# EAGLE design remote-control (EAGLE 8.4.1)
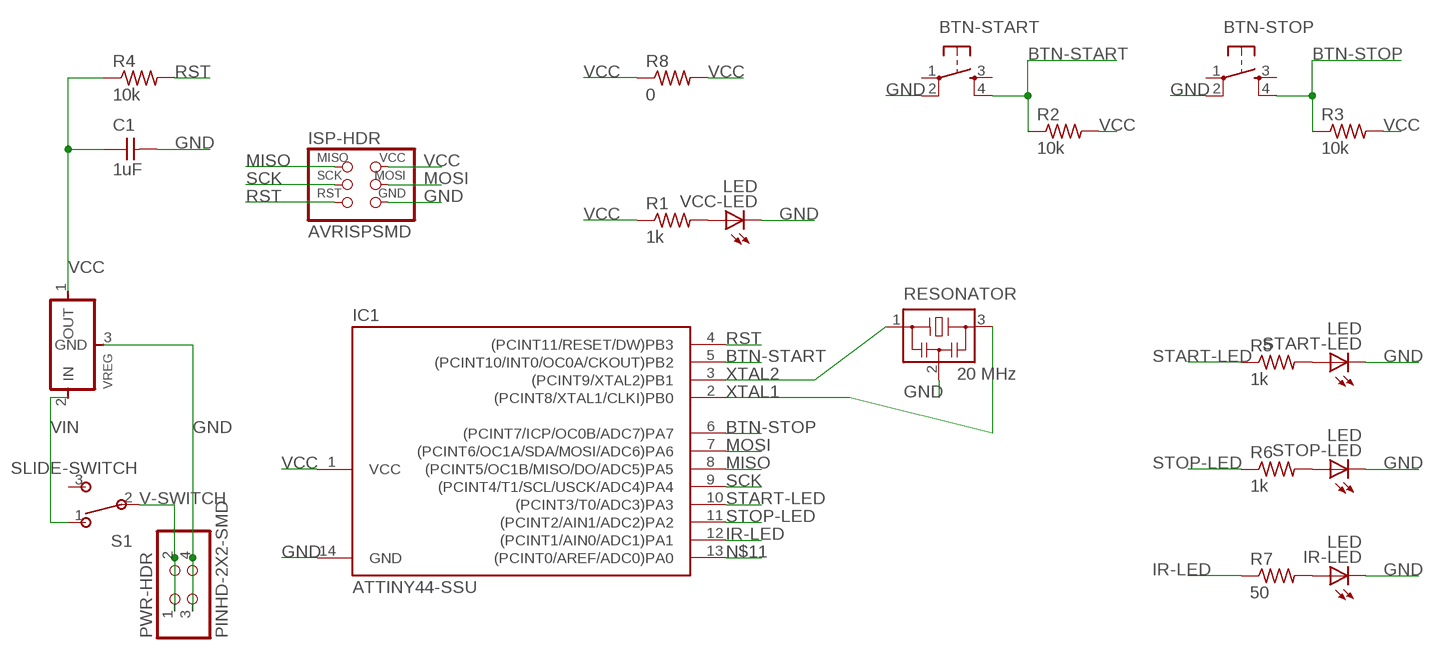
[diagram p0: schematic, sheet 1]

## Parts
BTN-START  6MM_SWITCH6MM_SWITCH  [6MM_SWITCH]
BTN-STOP  6MM_SWITCH6MM_SWITCH  [6MM_SWITCH]
C1  1uF  CAP-UNPOLARIZEDFAB  [C1206FAB]
IC1  ATTINY44-SSU  [SOIC14]
IR-LED  LED  [LED1206]
ISP-HDR  AVRISPSMD  [2X03SMD]
PWR-HDR  PINHD-2X2-SMD  [2X02SMD]
R1  1k  RES-US1206FAB  [R1206FAB]
R2  10k  RES-US1206FAB  [R1206FAB]
R3  10k  RES-US1206FAB  [R1206FAB]
R4  10k  RES-US1206FAB  [R1206FAB]
R5  1k  RES-US1206FAB  [R1206FAB]
R6  1k  RES-US1206FAB  [R1206FAB]
R7  50  RES-US1206FAB  [R1206FAB]
R8  0  RES-US1206FAB  [R1206FAB]
RESONATOR  20 MHz  RESONATOR  [EFOBM]
S1  SLIDE-SWITCH  [AYZ0102AGRLC]
START-LED  LED  [LED1206]
STOP-LED  LED  [LED1206]
VCC-LED  LED  [LED1206]
VREG  REGULATORSOT23  [SOT23]

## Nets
BTN-START: BTN-START.4(S1) IC1.5((PCINT10/INT0/OC0A/CKOUT)PB2) R2.1
BTN-STOP: BTN-STOP.4(S1) IC1.6((PCINT7/ICP/OC0B/ADC7)PA7) R3.1
GND: BTN-START.2(P1) BTN-STOP.2(P1) C1.2 IC1.14(GND) IR-LED.2(C) ISP-HDR.6(GND) PWR-HDR.3 PWR-HDR.4 RESONATOR.2 START-LED.2(C) STOP-LED.2(C) VCC-LED.2(C) VREG.3(GND)
IR-LED: IC1.12((PCINT1/AIN0/ADC1)PA1) R7.1
MISO: IC1.8((PCINT5/OC1B/MISO/DO/ADC5)PA5) ISP-HDR.1(MISO)
MOSI: IC1.7((PCINT6/OC1A/SDA/MOSI/ADC6)PA6) ISP-HDR.4(MOSI)
N$2: R5.2 START-LED.1(A)
N$3: R6.2 STOP-LED.1(A)
N$4: IR-LED.1(A) R7.2
N$9: R1.2 VCC-LED.1(A)
N$11: IC1.13((PCINT0/AREF/ADC0)PA0)
RST: IC1.4((PCINT11/RESET/DW)PB3) ISP-HDR.5(RST) R4.2
SCK: IC1.9((PCINT4/T1/SCL/USCK/ADC4)PA4) ISP-HDR.3(SCK)
START-LED: IC1.10((PCINT3/T0/ADC3)PA3) R5.1
STOP-LED: IC1.11((PCINT2/AIN1/ADC2)PA2) R6.1
V-SWITCH: PWR-HDR.1 PWR-HDR.2 S1.2
VCC: C1.1 IC1.1(VCC) ISP-HDR.2(VCC) R1.1 R2.2 R3.2 R4.1 R8.1 R8.2 VREG.1(OUT)
VIN: S1.1 VREG.2(IN)
XTAL1: IC1.2((PCINT8/XTAL1/CLKI)PB0) RESONATOR.3
XTAL2: IC1.3((PCINT9/XTAL2)PB1) RESONATOR.1
Unconnected: BTN-START.1(P) BTN-START.3(S) BTN-STOP.1(P) BTN-STOP.3(S) S1.3

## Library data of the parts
BTN-START BTN-STOP = fab:6MM_SWITCH: OMRON SWITCH
C1 = fab:CAP-UNPOLARIZED
IC1 = fab:ATTINY44
IR-LED START-LED STOP-LED VCC-LED = fab:LED: LED
ISP-HDR = fab:AVRISP
PWR-HDR = fab:PINHD-2X2-SMD
R1-R8 = fab:RES-US: Resistor (US Symbol)
RESONATOR = fab:RESONATOR
S1 = fab:SLIDE-SWITCH: SMD slide-switch AYZ0102AGRLC as found in the fablab inventory. Includes the mounting holes. Made by Zaerc.
VREG = fab:REGULATOR

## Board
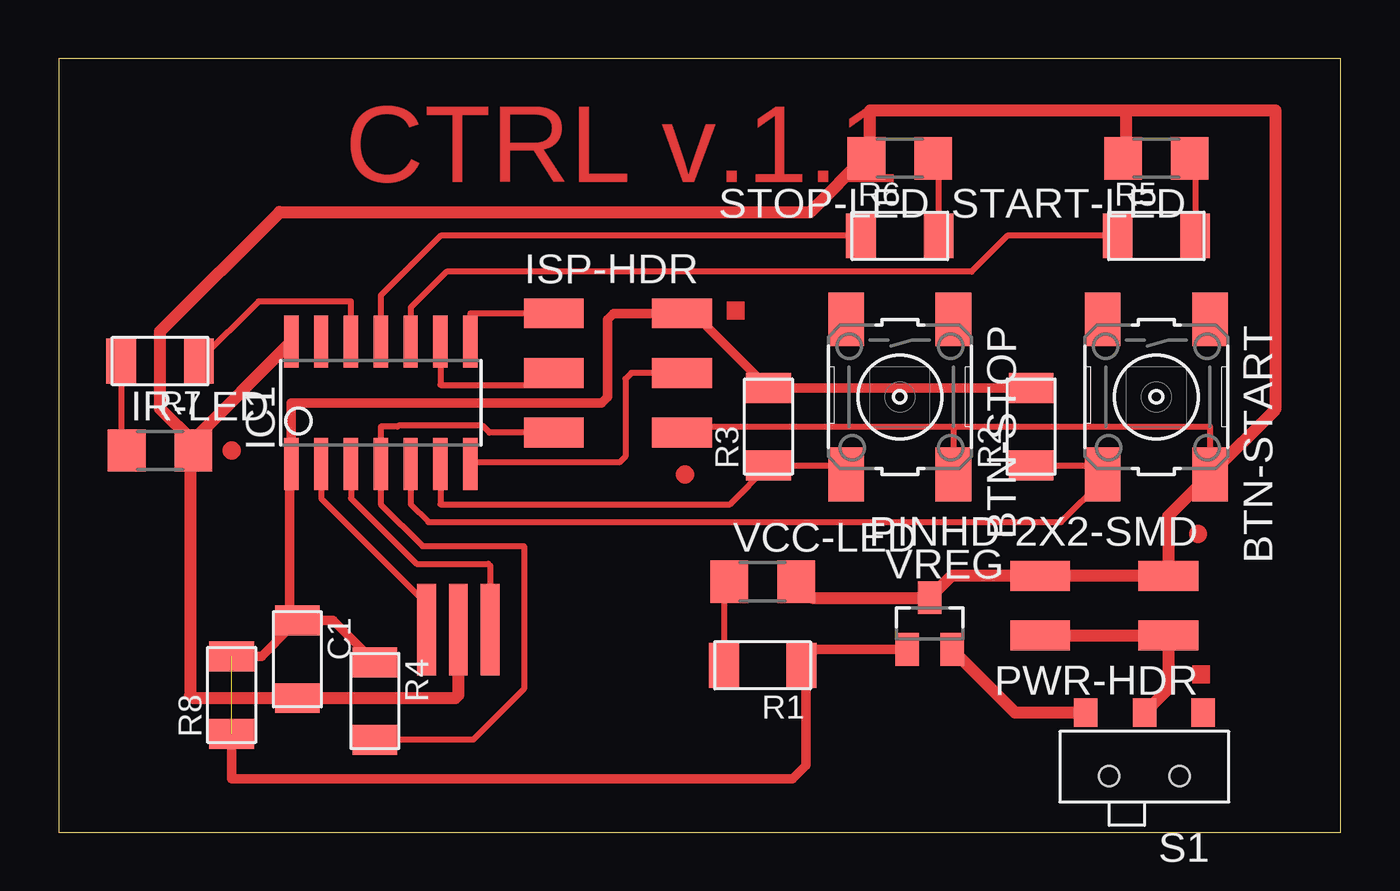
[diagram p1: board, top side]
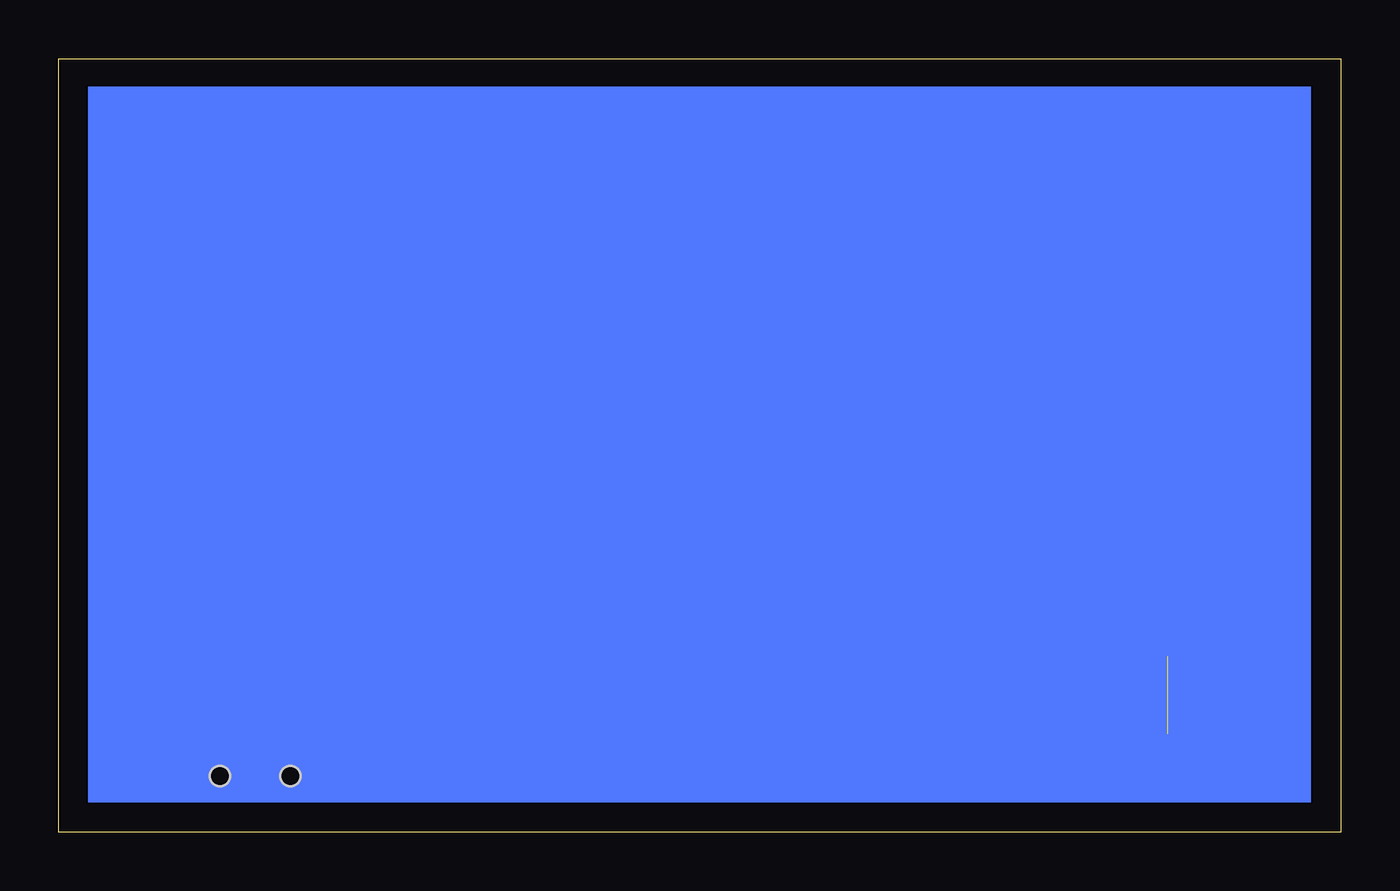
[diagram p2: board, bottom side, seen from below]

Size 54.59 x 32.94 mm. Coordinates in mm from the lower left corner, seen from the top.
Outline: 0,0 54.59,0 54.59,32.94 0,32.94 0,0
Copper layers (1*16): Top 0.035mm / dielectric 1.5mm / Bottom 0.035mm
Design rules "default *": minimum track width 0.000253125mm, minimum drill 0.35mm, track to track 15.625mil, track to pad 15.625mil, pad to pad 15.625mil, via to via 15.625mil, smd to smd 6mil, copper to edge 15.625mil, drill to drill 15.625mil, minimum pad ring 10mil, minimum via ring 8mil, stop-mask expansion 4mil, vias tented up to drill 0mil, thermal gap 10mil

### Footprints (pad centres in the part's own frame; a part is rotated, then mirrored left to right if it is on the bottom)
6MM_SWITCH = smd 2.286 x 1.524: 1 -3.302,2.286; 2 3.302,2.286; 3 -3.302,-2.286; 4 3.302,-2.286
C1206FAB = smd 1.27 x 1.905: 1 -1.651,0; 2 1.651,0
SOIC14 = smd 0.61 x 2.21: 1 -3.81,-2.603; 2 -2.54,-2.603; 3 -1.27,-2.603; 4 0,-2.603; 5 1.27,-2.603; 6 2.54,-2.603; 7 3.81,-2.603; 8 3.81,2.603; 9 2.54,2.603; 10 1.27,2.603; 11 0,2.603; 12 -1.27,2.603; 13 -2.54,2.603; 14 -3.81,2.603
LED1206 = smd 1.6 x 1.803: 1 -1.422,0; 2 1.422,0
2X03SMD = smd 2.54 x 1.27: 1 -2.54,2.54; 2 2.92,2.54; 3 -2.54,0; 4 2.92,0; 5 -2.54,-2.54; 6 2.92,-2.54
2X02SMD = smd 2.54 x 1.27: 1 -2.54,1.27; 2 2.92,1.27; 3 -2.54,-1.27; 4 2.92,-1.27
R1206FAB = smd 1.27 x 1.905: 1 -1.651,0; 2 1.651,0
EFOBM = smd 0.8 x 3.9: 1 -1.35,0; 2 0,0; 3 1.35,0
AYZ0102AGRLC = smd 1 x 1.2: 1 2.5,-2.3; 2 0,-2.3; 3 -2.5,-2.3 | hole 0.85: -1.5,0.4; 1.5,0.4
SOT23 = smd 1 x 1.4: 1 -0.95,-1.1; 2 0.95,-1.1; 3 0,1.1

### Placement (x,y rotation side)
BTN-START  46.74,18.54 270 top
BTN-STOP  35.81,18.54 270 top
C1  10.16,7.37 270 top
IC1  13.72,18.29 0 top
IR-LED  4.32,16.26 0 top
ISP-HDR  23.62,19.56 0 top
PWR-HDR  44.7,9.65 180 top
R1  29.97,7.11 180 top
R2  41.4,17.27 90 top
R3  30.23,17.27 90 top
R4  13.46,5.59 270 top
R5  46.74,25.4 0 top
R6  35.81,25.4 0 top
R7  4.32,20.07 180 top
R8  7.37,5.84 90 top
RESONATOR  17.02,8.64 180 top
S1  46.23,2.79 180 top
START-LED  46.74,28.7 180 top
STOP-LED  35.81,28.7 180 top
VCC-LED  29.97,10.67 0 top
VREG  37.08,8.89 0 top

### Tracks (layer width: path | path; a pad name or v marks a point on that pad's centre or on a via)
BTN-START
  Top 0.254: R2.1 44.07,15.62 BTN-START.4 44.45,14.99 42.67,13.21 15.75,13.21 14.99,13.97 IC1.5
BTN-STOP
  Top 0.254: IC1.6 16.26,13.97 28.57,13.97 R3.1 33.15,15.62 BTN-STOP.4
GND
  Top 0.254: VCC-LED.2 32.07,9.99 | ISP-HDR.6 26.8,17.27 38.1,17.27 | 38.1,17.27 BTN-STOP.2 | 38.1,17.27 49.02,17.27 49.02,15.49 49.28,15.24 | 5.74,16.61 IR-LED.2 5.59,16.1 | 34.44,28.85 34.54,28.85 | 5.71,5.71 5.59,5.84
  Top 0.508: 49.28,15.24 BTN-START.2 | START-LED.2 45.47,28.85 45.47,30.73 | 45.47,30.73 51.82,30.73 51.82,18.03 BTN-START.2 | 45.47,30.73 34.54,30.73 34.54,28.85 STOP-LED.2 | 32.07,9.99 VREG.3 38.02,10.92 PWR-HDR.4 PWR-HDR.3 47.24,13.46 BTN-START.2 | 5.74,16.61 4.32,18.03 4.32,21.34 9.4,26.42 32,26.42 34.44,28.85 | 5.71,5.71 C1.2 16.89,5.71 17.02,5.84 RESONATOR.2 | 5.59,5.84 5.59,16.1 5.59,16.57 IC1.14
IR-LED
  Top 0.254: IC1.12 12.45,22.61 8.51,22.61 R7.1
MISO
  Top 0.254: ISP-HDR.1 17.53,22.1 IC1.8 17.59,20.83
MOSI
  Top 0.254: ISP-HDR.4 24.38,19.56 24.13,19.3 24.13,16 23.88,15.75 17.59,15.75 IC1.7
N$2
  Top 0.254: START-LED.1 48.39,28.47 R5.2
N$3
  Top 0.254: STOP-LED.1 37.47,28.47 R6.2
N$4
  Top 0.254: R7.2 2.67,16.48 IR-LED.1
N$9
  Top 0.254: VCC-LED.1 28.32,10.44 R1.2
RST
  Top 0.254: ISP-HDR.5 18.34,17.02 18.05,17.31 14.46,17.31 14.42,17.27 13.72,17.27 IC1.4 13.72,13.97 15.49,12.19 19.81,12.19 19.81,6.1 17.65,3.94 R4.2
SCK
  Top 0.254: IC1.9 16.26,19.05 20.57,19.05 ISP-HDR.3
START-LED
  Top 0.254: R5.1 40.39,25.4 38.86,23.88 16.51,23.88 14.99,22.35 IC1.10
STOP-LED
  Top 0.254: IC1.11 13.72,22.86 16.26,25.4 R6.1
V-SWITCH
  Top 0.508: PWR-HDR.2 PWR-HDR.1 47.24,6.11 S1.2
VCC  (1 unrouted)
  Top 0.254: R1.1 31.81,7.3 32.3,7.79
  Top 0.406: 32.3,7.79 VREG.1 | R2.2 R3.2 27.05,22.1 ISP-HDR.2 23.62,22.1 23.37,21.84 23.37,18.54 23.11,18.29 9.91,18.29 IC1.1 9.84,15.62 9.84,8.7 | R8.2 8.64,7.49 9.84,8.7 | 9.84,8.7 C1.1 11.68,9.02 R4.1 | R8.1 7.37,2.29 31.24,2.29 31.81,2.86 31.81,7.3
VIN
  Top 0.508: S1.1 40.73,5.09 VREG.2
XTAL1
  Top 0.254: IC1.2 11.18,14.22 15.67,9.73 RESONATOR.3
XTAL2
  Top 0.254: IC1.3 12.45,14.22 15.24,11.43 18.29,11.43 18.37,11.35 RESONATOR.1
(copper drawn outside any net)
  shapes: Bottom area x1, Top area x2, Top circle x3

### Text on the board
Top: CTRL v.1.1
